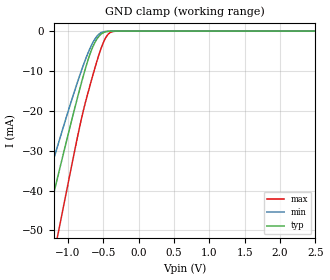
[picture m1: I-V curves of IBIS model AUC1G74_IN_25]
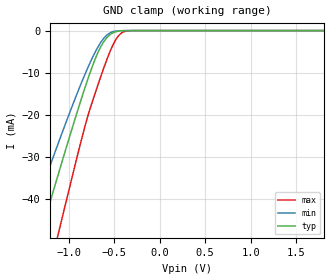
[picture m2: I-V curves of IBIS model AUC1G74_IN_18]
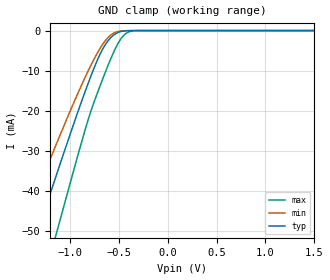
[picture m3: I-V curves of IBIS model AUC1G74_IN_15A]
| TEXAS INSTRUMENTS INCORPORATED
| Standard Linear and Logic Group
| IBIS Model of SN74AUC1G74
| DUAL POSITIVE-EDGE-TRIGGERED D-TYPE FLIP FLOP WITH CLEAR AND PRESET
| This file contains package information for the following:
|  SOT 8-pin (DCU) package as [Component] AUC1G74_DCU
|  TSSOP 8-pin (DCT) package as [Component] AUC1G74_DCT
|  NanoStar WCSP 8-pin (YEA) package as [Component] AUC1G74_YEA
|  NanoFree WCSP 8-pin (YZA) package as [Component] AUC1G74_YZA
| This device can be powered at the following Vccs:
|  2.5 volt Vcc
|  1.8 volt Vcc
|  1.5 volt Vcc
|  1.2 volt Vcc
|  0.8 volt Vcc
| This file provides unique models under the [Model Selector] for each Vcc.
| For operation at a specific Vcc, select the appropriate model after each
| [Model Selector] keyword.
[IBIS Ver]   3.2
[Comment char]  |_char
[File Name]   sn74auc1g74.ibs
[File Rev]   1.1 | x_die
[Date]   December 30, 2003
[Source]   Data created from TI-SPICE simulations at TI-SLL.
[Notes]   The following is an IBIS list for the AUC1G74.
   Please contact sllibis@ti.com with questions and
   comments concerning SLL IBIS models.
   -Power clamp data deleted as there is no power-clamp diode.
   -The waveforms for the AUC1G79_OUT Pullup, and
   Pulldown are caused by the circuitry that helps reduce
   overshoot and undershoot in transmission lines (EMI).
   These waveforms are normal for this particular design.
   -End point warning due to AC and DC mismatch.
[Disclaimer] Property of Texas Instruments Incorporated.  Unauthorized
   reproduction and/or distribution is strictly prohibited.
   This product is protected under copyright law.
   Created  2003, (C) Copyright  2003, Texas Instruments
   Incorporated, All Rights Reserved
   UNLESS THERE IS A SIGNED, WRITTEN AGREEMENT TO THE
   CONTRARY, TEXAS INSTRUMENTS (TI) IS PROVIDING THE IBIS
   MODELS  AND WITHOUT ANY WARRANTY, EXPRESSED OR
   IMPLIED.  TI assumes no liability for:
   1) the accuracy of the IBIS models provided to your
   company;
   2) the proper functioning of these IBIS Models in your
   design or for any resulting applications; or
   3) infringement of patents, copyrights or intellectual
   property rights resulting from your use of these IBIS
   models.
   TI provides IBIS Models as a service to our customers.
   You and your company shall not distribute, sell or give
   these models to anyone else without prior written
   permission from TI.
   TI reserves the right to make changes to our products or
   to discontinue any semiconductor product or service
   without notice, and advises our customers to obtain the
   latest version of relevant information to verify, before
   placing orders, that the information being relied on is
   current.
   Please be aware that your receipt and use of the IBIS
   information provided shall serve as acceptance of these
   terms and conditions.  If you do not accept these terms,
   you should return or destroy the IBIS models and any
   other accompanying information immediately.
| Component AUC1G74_DCU 8-pin SOT
[Component]   AUC1G74_DCU
[Manufacturer]   Texas Instruments, Inc.
[Package]
|   typ   min   max
R_pkg   2.600e-02   2.300e-02   3.800e-02
L_pkg   1.394e-09   1.066e-09   2.046e-09
C_pkg   2.590e-13   2.150e-13   3.720e-13
[Pin]   signal_name   model_name   R_pin   L_pin   C_pin
1   CLK   AUC1G74_IN   2.400e-02   1.520e-09   2.710e-13
2   DIN   AUC1G74_IN   2.300e-02   1.112e-09   2.180e-13
3   QB   AUC1G74_OUT   2.300e-02   1.070e-09   2.170e-13
4   GND   GND   2.700e-02   2.046e-09   3.720e-13
5   Q   AUC1G74_OUT   2.700e-02   1.542e-09   2.730e-13
6   CLRZ   AUC1G74_IN   2.300e-02   1.100e-09   2.240e-13
7   PREZ   AUC1G74_IN   2.300e-02   1.066e-09   2.150e-13
8   VCC   POWER   3.800e-02   1.696e-09   2.800e-13
| Component AUC1G74_DCT 8-pin TSSOP
[Component]   AUC1G74_DCT
[Manufacturer]   Texas Instruments, Inc.
[Package]
|   typ   min   max
R_pkg   2.900e-02   2.800e-02   3.100e-02
L_pkg   1.796e-09   1.666e-09   1.924e-09
C_pkg   1.090e-13   8.300e-14   1.360e-13
[Pin]   signal_name   model_name   R_pin   L_pin   C_pin
1   CLK   AUC1G74_IN   3.100e-02   1.894e-09   1.340e-13
2   DIN   AUC1G74_IN   2.800e-02   1.697e-09   8.600e-14
3   QB   AUC1G74_OUT   3.000e-02   1.722e-09   8.600e-14
4   GND   GND   3.000e-02   1.861e-09   1.300e-13
5   Q   AUC1G74_IN   2.800e-02   1.924e-09   1.360e-13
6   CLRZ   AUC1G74_OUT   2.900e-02   1.736e-09   8.600e-14
7   PREZ   AUC1G74_IN   2.800e-02   1.666e-09   8.300e-14
8   VCC   POWER   3.000e-02   1.871e-09   1.320e-13
| Component AUC1G74_YEP 8-pin NanoStar WCSP
[Component]   AUC1G74_YEP
[Manufacturer]   Texas Instruments, Inc.
[Package]
|   typ   min   max
R_pkg   0.001   0.001   0.001
L_pkg   0.021nH   0.021nH   0.021nH
C_pkg   0.043pF   0.042pF   0.044pF
[Pin]   signal_name   model_name   R_pin   L_pin   C_pin
1   CLK   AUC1G74_IN   0.046   2.861nH   0.321pF
2   D   AUC1G74_IN   0.037   2.437nH   0.286pF
3   NQ   AUC1G74_OUT   0.034   2.419nH   0.286pF
4   GND   GND   0.043   2.784nH   0.321pF
5   Q   AUC1G74_IN   0.043   2.784nH   0.321pF
6   NCLR   AUC1G74_IN   0.035   2.420nH   0.286pF
7   NPRE   AUC1G74_OUT   0.037   2.437nH   0.286pF
8   VCC   POWER   0.046   2.860nH   0.321pF
| Component AUC1G74_YZP 8-pin NanoFree WCSP
[Component]   AUC1G74_YZP
[Manufacturer]   Texas Instruments, Inc.
[Package]
|   typ   min   max
R_pkg   0.001   0.001   0.001
L_pkg   0.021nH   0.021nH   0.021nH
C_pkg   0.043pF   0.042pF   0.044pF
[Pin]   signal_name   model_name   R_pin   L_pin   C_pin
1   CLK   AUC1G74_IN   0.046   2.861nH   0.321pF
2   D   AUC1G74_IN   0.037   2.437nH   0.286pF
3   NQ   AUC1G74_OUT   0.034   2.419nH   0.286pF
4   GND   GND   0.043   2.784nH   0.321pF
5   Q   AUC1G74_IN   0.043   2.784nH   0.321pF
6   NCLR   AUC1G74_IN   0.035   2.420nH   0.286pF
7   NPRE   AUC1G74_OUT   0.037   2.437nH   0.286pF
8   VCC   POWER   0.046   2.860nH   0.321pF
| Model AUC1G74_IN
[Model Selector]   AUC1G74_IN
AUC1G74_IN_25   2.5 volt Vcc
AUC1G74_IN_18   1.8 volt Vcc
AUC1G74_IN_15A   1.5 volt Vcc
AUC1G74_IN_12   1.2 volt Vcc
AUC1G74_IN_08   0.8 volt Vcc
| Model AUC1G74_OUT
[Model Selector]   AUC1G74_OUT
AUC1G74_OUT_25   2.5 volt Vcc
AUC1G74_OUT_18   1.8 volt Vcc
AUC1G74_OUT_15A   1.5 volt Vcc
AUC1G74_OUT_12   1.2 volt Vcc
AUC1G74_OUT_08   0.8 volt Vcc
| Models and submodels in the file (10): AUC1G74_IN_25 (Input), AUC1G74_IN_18 (Input), AUC1G74_IN_15A (Input), AUC1G74_IN_12 (Input), AUC1G74_IN_08 (Input), AUC1G74_OUT_25 (Output), AUC1G74_OUT_18 (Output), AUC1G74_OUT_15A (Output), AUC1G74_OUT_12 (Output), AUC1G74_OUT_08 (Output)
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[Model]   AUC1G74_IN_25
Model_type  Input
Vinl=0.7
Vinh=1.7
| variable   typ   min   max
C_comp   2.45pF   1.97pF   2.83pF
[Temperature Range]   40   100   -40
| Ambient temperature   25   85   -40
[Voltage range]   2.5   2.3   2.7
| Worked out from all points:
|   GND clamp passes 1 mA (typ) near -0.55 V on its own axis
[GND Clamp]
| AUC1G74_IN_25
|   Voltage   I(typ)   I(min)   I(max)
-3.6V     -222.3mA   -186mA     -267.4mA
-1.49V    -62.27mA   -49.76mA   -82.08mA
-1.35V    -51.78mA   -41.12mA   -69.61mA
-1.305V   -48.43mA   -38.37mA   -65.59mA
-1.17V    -38.45mA   -30.23mA   -53.54mA
-1.12V    -34.78mA   -27.27mA   -49.07mA
-735mV    -8.323mA   -6.326mA   -16.67mA
-635mV    -3.426mA   -2.469mA   -10.25mA
-525mV    -682.5uA   -360.1uA   -4.021mA
-430mV    -73.19uA   -34.72uA   -776.9uA
-325mV    -3.339uA   -2.005uA   -30.74uA
2.5V      313.9pA    400.8pA    470.4pA
[Model]   AUC1G74_IN_18
Model_type  Input
Vinl=0.5775
Vinh=1.2675
| variable   typ   min   max
C_comp   2.51pF   2.06pF   2.87pF
[Temperature Range]   40   100   -40
| Ambient temperature   25   85   -40
[Voltage range]   1.8   1.65   1.95
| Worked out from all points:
|   GND clamp passes 1 mA (typ) near -0.55 V on its own axis
[GND Clamp]
| AUC1G74_IN_18
|   Voltage   I(typ)   I(min)   I(max)
-3.6V     -222.3mA   -186mA     -267.4mA
-1.475V   -61.14mA   -48.83mA   -80.75mA
-1.43V    -57.76mA   -46.04mA   -76.74mA
-1.295V   -47.69mA   -37.76mA   -64.7mA
-1.1V     -33.32mA   -26.09mA   -47.29mA
-830mV    -14.31mA   -10.95mA   -23.64mA
-680mV    -5.361mA   -4.028mA   -13.09mA
-560mV    -1.272mA   -753.1uA   -5.827mA
-485mV    -290.6uA   -140.1uA   -2.305mA
-420mV    -55.81uA   -26.71uA   -608.5uA
-300mV    -1.501uA   -987.4nA   -11.88uA
1.8V      203.2pA    297.2pA    235.5pA
[Model]   AUC1G74_IN_15A
Model_type  Input
Vinl=0.49
Vinh=1.04
| variable   typ   min   max
C_comp   2.54pF   2.10pF   2.86pF
[Temperature Range]   40   100   -40
| Ambient temperature   25   85   -40
[Voltage range]   1.5   1.4   1.6
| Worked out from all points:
|   GND clamp passes 1 mA (typ) near -0.55 V on its own axis
[GND Clamp]
| AUC1G74_IN_15A
|   Voltage   I(typ)   I(min)   I(max)
-3.6V     -222.3mA   -186mA     -267.4mA
-1.505V   -63.39mA   -50.69mA   -83.42mA
-1.325V   -49.92mA   -39.59mA   -67.38mA
-1.17V    -38.45mA   -30.23mA   -53.54mA
-1.12V    -34.78mA   -27.27mA   -49.07mA
-840mV    -14.97mA   -11.47mA   -24.46mA
-695mV    -6.113mA   -4.618mA   -14.06mA
-570mV    -1.487mA   -910.9uA   -6.381mA
-495mV    -364.6uA   -178.7uA   -2.692mA
-430mV    -73.19uA   -34.72uA   -776.9uA
-280mV    -781.4nA   -556.2nA   -5.358uA
1.5V      165.9pA    258.5pA    172.1pA
